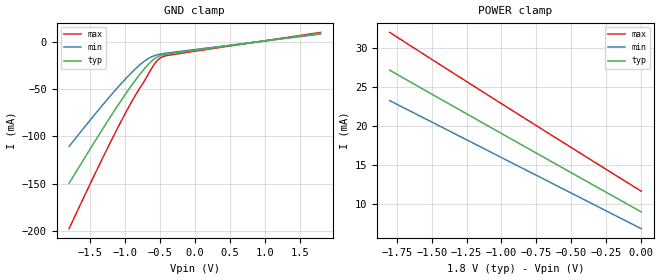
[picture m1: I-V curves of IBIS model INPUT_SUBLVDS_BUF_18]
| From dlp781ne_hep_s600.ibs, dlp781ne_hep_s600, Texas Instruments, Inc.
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[Model]   INPUT_SUBLVDS_BUF_18
Model_type  Input
Vinl=0.80
Vinh=1.00
| variable   typ   min   max
C_comp   0.69pF   0.66pF   0.72pF
[Temperature Range]   25   85   -40
[Voltage range]   1.8   1.65   1.95
[GND Clamp]
| INPUT_SUBLVDS_BUF_18
|   Voltage   I(typ)   I(min)   I(max)
-1.8V     -149.7mA   -110.7mA   -197.8mA
-1.29V    -88.84mA   -64.29mA   -118.6mA
-1.095V   -66.55mA   -47.56mA   -89.83mA
-930mV    -48.67mA   -34.42mA   -66.87mA
-790mV    -34.7mA    -24.56mA   -49.3mA
-680mV    -25.03mA   -18.39mA   -35.98mA
-580mV    -18.08mA   -14.73mA   -23.73mA
-510mV    -15.09mA   -13.26mA   -17.94mA
-450mV    -13.75mA   -12.43mA   -15.53mA
-355mV    -12.57mA   -11.45mA   -13.96mA
1.8V      8.993mA    8.203mA    9.976mA
[POWER Clamp]
| INPUT_SUBLVDS_BUF_18
|   Voltage   I(typ)   I(min)   I(max)
-1.8V     27.16mA    23.26mA    32.02mA
-1.37V    22.79mA    19.34mA    27.08mA
-920mV    18.24mA    15.23mA    21.97mA
-16.28fV  8.993mA    6.835mA    11.65mA
